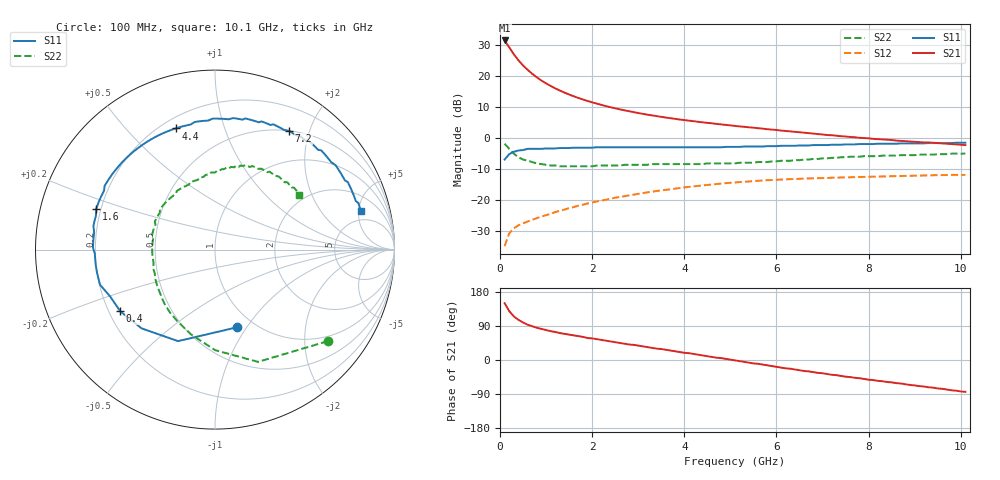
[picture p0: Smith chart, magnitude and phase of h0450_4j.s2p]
!HBFP-0450
!S and NOISE PARAMETERS at Vce=4V  Ic=100mA.  LAST UPDATED  09-04-98
# GHZ S MA R  50
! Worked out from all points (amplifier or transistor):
!   101 points, 100 MHz to 10.1 GHz, reference 50 ohm
!   highest |S21| = 31.5 dB at 100 MHz (marker M1)
!   |S21| within 3 dB of that: start of sweep to 234.8 MHz
!   unconditionally stable (mu >= 1): 2.18 GHz to end of sweep
!   at 1.7 GHz: K = 0.95, MSG = 17.4 dB, |S12| = -21.8 dB
!   at 5.1 GHz: K = 1.08, MAG = 7.4 dB, |S12| = -14.3 dB
!   at 10.1 GHz: K = 1.06, MAG = 3.3 dB, |S12| = -11.9 dB
!   lowest NFmin = 2.38 dB at 1.8 GHz
!   S11 on the Smith chart (normalised r, x): 100 MHz: 0.84, -0.91; 400 MHz: 0.25, -0.28; 1.6 GHz: 0.18, +0.16; 4.4 GHz: 0.26, +0.70; 7.2 GHz: 0.50, +1.69; 10.1 GHz: 3.55, +5.25
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0.1  0.45 -74.0  37.57 150.0  0.018 62.0  0.81 -39.0
0.2  0.55 -112.0  29.08 129.0  0.029 50.0  0.67 -69.0
0.3  0.6 -133.0  22.5 115.0  0.035 45.0  0.56 -90.0
0.4  0.63 -147.0  17.98 106.0  0.039 42.0  0.49 -106.0
0.5  0.64 -156.0  14.81 99.0  0.042 41.0  0.45 -118.0
0.6  0.67 -163.0  12.61 93.0  0.045 40.0  0.43 -126.0
0.7  0.67 -169.0  10.87 89.0  0.048 41.0  0.41 -134.0
0.8  0.67 -173.0  9.53 85.0  0.051 41.0  0.39 -142.0
0.9  0.67 -178.0  8.47 82.0  0.054 42.0  0.38 -148.0
1  0.68 179.0  7.62 79.0  0.057 42.0  0.37 -154.0
1.2  0.68 172.0  6.33 74.0  0.064 43.0  0.36 -163.0
1.4  0.69 167.0  5.41 69.0  0.07 43.0  0.35 -172.0
1.6  0.7 161.0  4.72 65.0  0.077 42.0  0.35 -179.0
1.8  0.7 157.0  4.19 61.0  0.084 41.0  0.35 175.0
2.5  0.71 142.0  3.02 47.0  0.109 36.0  0.36 159.0
3.5  0.71 124.0  2.2 29.0  0.143 26.0  0.38 141.0
4.4  0.71 108.0  1.79 12.0  0.172 14.0  0.38 125.0
5.1  0.72 95.0  1.57 -1.0  0.192 4.0  0.39 112.0
6.8  0.77 65.0  1.18 -32.0  0.224 -21.0  0.46 82.0
7.2  0.78 58.0  1.11 -39.0  0.229 -27.0  0.48 76.0
8.5  0.81 38.0  0.93 -59.0  0.242 -44.0  0.52 58.0
10.1  0.84 15.0  0.77 -84.0  0.254 -67.0  0.56 33.0
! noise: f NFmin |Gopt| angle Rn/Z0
1.8  2.38  0.68  -147  0.17
2  2.45  0.67  -145  0.2
2.5  2.6  0.67  -135  0.31
3.5  2.92  0.7  -119  0.6
4  3.07  0.72  -109  0.86
5  3.39  0.73  -90  1.46
5.5  3.55  0.75  -81  1.96
7  4.02  0.78  -55  3.72
8  4.33  0.81  -39  5.29
10  4.96  0.83  -11  8.06
